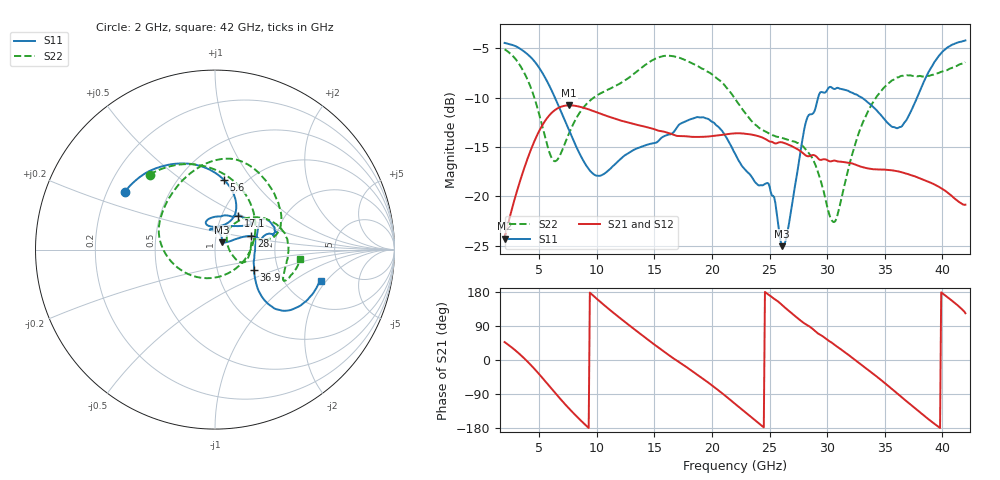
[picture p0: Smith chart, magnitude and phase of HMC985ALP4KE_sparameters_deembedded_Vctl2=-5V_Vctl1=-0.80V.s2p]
!s2p File: Measurements: S11, S21, S12, S22
# GHz S dB R 50.0
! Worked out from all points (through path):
!   401 points, 2 GHz to 42 GHz, reference 50 ohm
!   highest |S21| = -10.79 dB at 7.6 GHz (marker M1); lowest = -24.3 dB at 2 GHz (marker M2)
!   lowest |S11| = -25.0 dB at 26.1 GHz (marker M3), VSWR 1.12, Z = 53.9 + j4.37 ohm
!   |S11| at or under -10 dB: 6.363 GHz to 29.22 GHz (22.85 GHz wide, 128 % of centre); 33.01 GHz to 37.81 GHz (4.8 GHz wide, 13.6 % of centre)
!   |S22| runs from -22.6 to -5.1 dB; largest |S21 - S12| = 0.00028
!   S11 on the Smith chart (normalised r, x): 2 GHz: 0.27, +0.27; 5.6 GHz: 0.81, +0.74; 17.1 GHz: 1.19, +0.48; 28 GHz: 1.49, +0.24; 36.9 GHz: 1.50, -0.36; 42 GHz: 3.12, -1.76
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2  -4.47 147.5  -24.27 47.2  -24.27 47.3  -5.12 131.1
3.6  -5.27 120.9  -17.50 7.3  -17.51 7.3  -7.27 86.1
4.7  -6.50 100.0  -14.11 -27.1  -14.12 -27.1  -10.46 44.4
5.6  -8.17 82.4  -12.21 -58.6  -12.22 -58.6  -14.39 -5.7
6.4  -10.10 69.4  -11.24 -87.3  -11.24 -87.3  -16.44 -69.1
7.6  -13.34 60.2  -10.79 -128.3  -10.79 -128.3  -13.60 -141.9
8.7  -16.11 66.5  -10.98 -162.2  -10.98 -162.2  -11.22 -174.3
12  -16.28 109.2  -12.30 111.1  -12.30 111.1  -8.59 137.8
15.4  -14.34 78.0  -13.36 31.9  -13.37 31.9  -5.93 86.2
17.1  -12.80 55.8  -13.89 -4.4  -13.89 -4.3  -5.96 66.1
19.6  -12.13 35.5  -13.95 -57.8  -13.95 -57.8  -7.37 32.3
22  -15.66 52.8  -13.62 -115.4  -13.63 -115.4  -10.12 11.2
24.9  -18.69 99.0  -14.38 172.6  -14.39 172.6  -13.60 11.9
26.1  -25.03 46.2  -14.54 144.7  -14.54 144.7  -14.09 -1.2
28  -13.27 20.4  -15.73 97.1  -15.74 97.1  -15.05 -23.4
28.7  -11.66 10.8  -15.83 83.1  -15.83 83.1  -16.10 -26.4
30.7  -9.12 18.6  -16.39 38.9  -16.39 38.9  -22.51 25.1
32.9  -9.94 32.2  -16.98 -11.1  -16.99 -11.1  -13.10 48.9
35.4  -12.72 10.0  -17.33 -70.8  -17.34 -70.8  -8.50 20.6
36.9  -12.24 -27.5  -17.70 -109.0  -17.71 -109.0  -7.74 2.6
39.6  -5.95 -42.4  -18.96 -174.9  -18.97 -174.8  -7.55 -24.2
42  -4.23 -16.6  -20.84 123.4  -20.84 123.4  -6.42 -6.2
